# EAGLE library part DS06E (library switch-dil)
DIL/CODE SWITCH
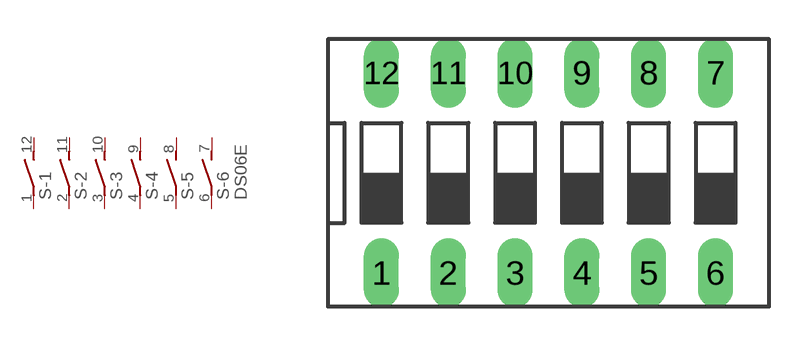
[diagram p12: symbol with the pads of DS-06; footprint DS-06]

Designator prefix S; gates -1=S -2=S -3=S -4=S -5=S -6=S+V

## DS06E (MPN: MCDS06; OC_FARNELL: 9471588; OC_NEWARK: 26M1105)  [DS-06]
1  -1:1  pas
2  -2:1  pas
3  -3:1  pas
4  -4:1  pas
5  -5:1  pas
6  -6:1  pas
7  -6:2  pas
8  -5:2  pas
9  -4:2  pas
10  -3:2  pas
11  -2:2  pas
12  -1:2  pas

## Footprint DS-06 (pad centres in mm)
DIL/CODE SWITCH Mors distributor Buerklin, 17G558
drill 0.813 long: 1 -6.35,-3.81; 2 -3.81,-3.81; 3 -1.27,-3.81; 4 1.27,-3.81; 5 3.81,-3.81; 6 6.35,-3.81; 7 6.35,3.81; 8 3.81,3.81; 9 1.27,3.81; 10 -1.27,3.81; 11 -3.81,3.81; 12 -6.35,3.81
